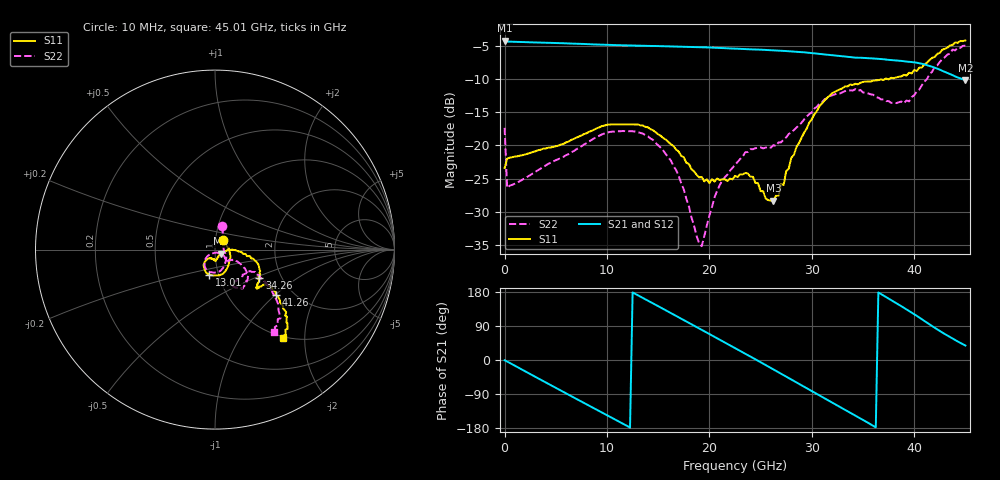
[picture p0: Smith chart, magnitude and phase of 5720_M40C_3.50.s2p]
! Device:  ADRF5720
! Description: 0.5dB LSB GaAs MMIC 6-bit Digital Attenuator
! Frequency:  0.000009 -  40 GHz
! Ports:
!	RF1	= Port 1
!	RF2	= Port 2
! Vdd:  3.3 Volt
! Vss:  -3.3 Volt
! Control:  0/3.3 Volt
! State:  3.50 dB attenuation
! Data:  The device was measured using G-S-G Probes on a matrix board.
!  Data was collected using an calibrated 4 port network analyzer.
!  The reference plane for this measurement is at the launchers.
! Note:  Analog Devices supplies this data as a sample of measured data
!  for this product.  Your particular data for this product may vary.
!  Data was taken at -40 degrees C.
!  Analog Devices reserves the right to change this data at anytime.
# GHZ S DB R 45.0
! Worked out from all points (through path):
!   181 points, 10 MHz to 45.01 GHz, reference 45 ohm
!   highest |S21| = -4.19 dB at 10 MHz (marker M1); lowest = -10.1 dB at 45.01 GHz (marker M2)
!   group delay of S21, straight-line fit = 41.8 ps
!   lowest |S11| = -28.4 dB at 26.26 GHz (marker M3), VSWR 1.08, Z = 47.9 - j2.09 ohm
!   |S11| at or under -10 dB: start of sweep to 37.14 GHz; 37.44333 GHz to 37.54846 GHz (105.1 MHz wide, 0.28 % of centre)
!   |S22| runs from -35.2 to -4.9 dB; largest |S21 - S12| = 0.0022
!   S11 on the Smith chart (normalised r, x): 10 MHz: 1.08, +0.11; 13.01 GHz: 0.90, -0.26; 34.26 GHz: 1.55, -0.53; 41.26 GHz: 1.64, -1.00; 45.01 GHz: 0.98, -1.57
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0.01  -23.42 51.1  -4.19 -0.7  -4.20 -0.7  -17.35 72.3
0.26  -22.00 1.7  -4.32 -4.0  -4.33 -4.1  -26.40 3.8
2.01  -21.37 -13.8  -4.40 -29.8  -4.42 -29.9  -24.94 -15.3
4.26  -20.35 -26.7  -4.51 -62.6  -4.53 -62.6  -22.80 -29.6
7.76  -18.29 -54.8  -4.68 -113.3  -4.70 -113.4  -19.87 -58.8
10.51  -16.81 -77.8  -4.84 -152.9  -4.85 -153.0  -17.92 -83.5
13.01  -16.83 -103.4  -4.94 171.1  -4.95 171.0  -18.00 -108.0
15.26  -18.56 -121.2  -5.00 138.3  -5.02 138.3  -20.36 -128.1
17.01  -20.92 -130.0  -5.07 112.8  -5.09 112.7  -24.62 -139.0
19.26  -24.77 -121.9  -5.17 79.6  -5.19 79.5  -35.22 -78.4
20.76  -25.01 -99.3  -5.26 57.4  -5.28 57.3  -26.86 -33.3
22.76  -24.78 -93.2  -5.40 27.7  -5.42 27.6  -22.47 -39.9
24.26  -24.75 -82.9  -5.50 5.4  -5.52 5.3  -20.58 -44.6
26.26  -28.37 -34.8  -5.64 -24.7  -5.66 -24.9  -19.96 -35.6
28.26  -21.43 -1.2  -5.83 -55.2  -5.85 -55.3  -17.69 -28.5
30.26  -15.30 -8.1  -6.09 -86.0  -6.11 -86.1  -14.44 -32.0
32.01  -12.10 -17.8  -6.39 -112.6  -6.41 -112.7  -12.44 -40.1
34.26  -10.69 -32.2  -6.74 -146.5  -6.76 -146.6  -11.50 -54.5
37.76  -9.78 -41.6  -7.11 158.2  -7.13 158.0  -13.59 -58.9
39.51  -9.02 -34.2  -7.38 129.5  -7.40 129.3  -13.35 -34.9
41.26  -7.52 -36.5  -7.89 98.4  -7.91 98.2  -9.97 -31.8
45.01  -4.15 -52.3  -10.11 38.1  -10.14 38.0  -4.94 -54.5
